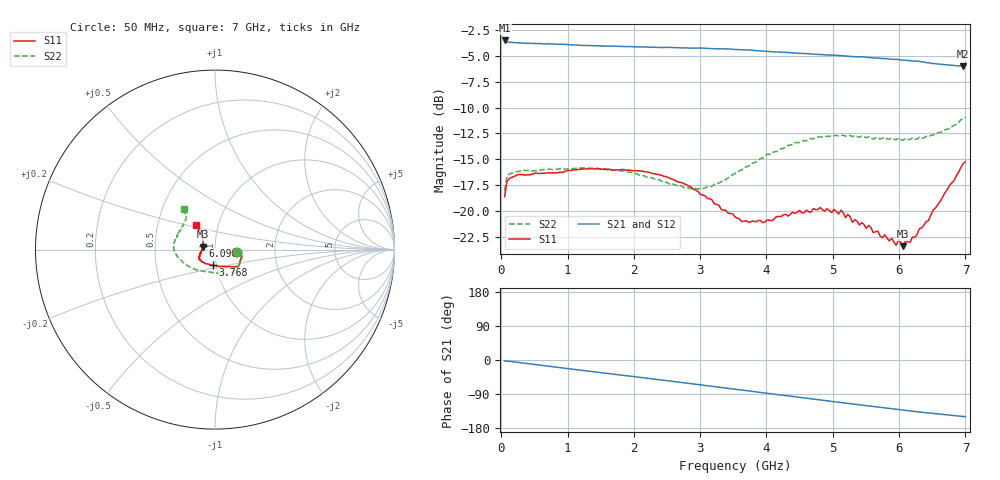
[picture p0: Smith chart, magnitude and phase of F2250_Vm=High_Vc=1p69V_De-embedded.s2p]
! Integrated Device Technology
! Corporate Headquarters
! 6024 Silver Creek Valley Road
! San Jose, CA 95138  USA
! Phone:  1-408-284-8200
! Toll Free:  1-800-223-1366
! Webpage:  http://www.idt.com/
! Timing and RF Division
! 515 Groton Road, Suite 102
! Westford, MA 01886-6024
! Device:  F2250
! Description: Voltage Variable RF Attenuator
! Frequency:  50.0 -  6000.00 MHz
! Package:  3x3 mm Thin QFN Plastic Package: 16 pin
! Ports:  2 RF, 3 DC
!  Pin  1  = GND
!  Pin  2  = NC
!  Pin  3  = RF1  = Port 1
!  Pin  4  = NC
!  Pin  5  = GND
!  Pin  6  = GND
!  Pin  7  = GND
!  Pin  8  = GND
!  Pin  9  = NC
!  Pin 10  = RF2  = Port 2
!  Pin 11  = NC
!  Pin 12  = GND
!  Pin 13  = GND
!  Pin 14  = VCNTRL
!  Pin 15  = VDD
!  Pin 16  = VMODE
! Vcntrl:  1.690 Volts
! Vmode:  +3.300 Volts
! Vdd:  +3.30  Volts
! Current:  1.326 mA
! Data:  The device was measured on a the F2250 evaluation board which has
!  individual transmission lines to the RF pins.  Data was collected
!  using a calibrated network analyzer.  The evaluation board was
!  de-embedded using a TRL calibration technique.
!  The reference plane is the edge of the package pin.
! Misc:  SN 10
!  Action Tracker AT0258
! Date Measured:  2014-11-26
! Date:  2015-10-15  MJV
! Note:
!  Integrated Device Technology supplies this data as a sample of measured
!  data at the package pin for this product.  Your particular data for this
!  product may vary.
!  Data was taken at 25 degrees C.
!  Integrated Device Technology reserves the right to change this data at anytime.
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# GHz S dB R 50
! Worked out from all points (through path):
!   201 points, 50 MHz to 7 GHz, reference 50 ohm
!   highest |S21| = -3.51 dB at 50 MHz (marker M1); lowest = -6.0 dB at 6.965 GHz (marker M2)
!   group delay of S21, straight-line fit = 60 ps
!   lowest |S11| = -23.4 dB at 6.062 GHz (marker M3), VSWR 1.14, Z = 43.8 + j1.46 ohm
!   |S11| at or under -10 dB: start of sweep to end of sweep
!   |S22| runs from -18.0 to -10.9 dB; largest |S21 - S12| = 0.0032
!   S11 on the Smith chart (normalised r, x): 50 MHz: 1.26, -0.03; 3.768 GHz: 0.96, -0.17; 6.096 GHz: 0.87, +0.04; 7 GHz: 0.78, +0.22
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0.05  -18.63 -6.1  -3.51 -2.4  -3.50 -2.4  -18.04 -7.1
0.08475  -17.18 -4.5  -3.63 -2.8  -3.64 -2.8  -16.69 -5.6
0.2585  -16.48 -8.4  -3.74 -6.5  -3.78 -6.5  -16.19 -11.6
1.2315  -15.95 -30.8  -3.98 -27.6  -3.97 -27.7  -15.84 -45.0
2.37825  -16.49 -39.5  -4.18 -51.9  -4.19 -51.9  -16.97 -71.7
2.969  -18.14 -49.3  -4.25 -64.9  -4.24 -64.9  -17.89 -98.4
3.525  -20.58 -78.3  -4.38 -77.3  -4.40 -77.4  -16.39 -131.8
3.76825  -21.04 -98.1  -4.45 -82.8  -4.48 -82.8  -15.46 -144.2
4.7065  -19.78 -145.5  -4.82 -103.3  -4.84 -103.3  -13.02 -176.1
5.1235  -19.93 -155.9  -4.98 -112.3  -4.98 -112.4  -12.70 173.6
5.29725  -21.11 -158.3  -5.06 -115.9  -5.06 -116.0  -12.81 170.0
5.5405  -21.41 -168.6  -5.15 -121.2  -5.14 -121.3  -12.82 163.3
5.85325  -22.91 180.0  -5.30 -127.7  -5.27 -127.9  -13.06 154.8
5.888  -22.65 179.7  -5.32 -128.5  -5.29 -128.6  -12.94 154.9
5.9575  -23.33 172.5  -5.33 -129.9  -5.32 -130.1  -13.11 152.1
5.99225  -22.80 170.3  -5.35 -130.8  -5.34 -130.9  -12.96 151.7
6.06175  -23.42 165.8  -5.41 -132.1  -5.40 -132.2  -13.16 149.0
6.0965  -22.93 162.5  -5.42 -133.0  -5.42 -133.1  -12.99 148.4
6.166  -23.03 157.3  -5.46 -134.4  -5.47 -134.4  -13.09 145.7
6.444  -20.94 138.3  -5.67 -140.0  -5.68 -140.1  -12.80 137.0
6.96525  -15.44 128.0  -6.01 -148.9  -6.01 -149.0  -11.07 128.8
7  -15.23 127.8  -6.00 -149.4  -6.01 -149.5  -10.93 128.0
